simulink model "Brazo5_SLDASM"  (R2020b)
settings: Solver=VariableStepAuto  StartTime=0.0  StopTime=10.0  RelTol=1e-3
undefined symbols (not defined in the file or in its folder): deg, kg, m, N, rad, s, X, Y, Z
libraries: sm_lib x59, nesl_utility x1

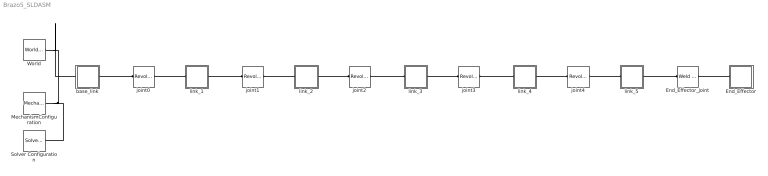
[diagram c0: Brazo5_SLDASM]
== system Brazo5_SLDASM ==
  End_Effector : Subsystem
  End_Effector_joint : sm_lib/Joints/Weld Joint  JointMode=Normal  SenseConstraintForce=off  SenseConstraintForceX=off  SenseConstraintForceY=off  SenseConstraintForceZ=off  SenseConstraintTorque=off  SenseConstraintTorqueX=off  SenseConstraintTorqueY=off  SenseConstraintTorqueZ=off  SenseTotalForce=off  SenseTotalForceX=off  SenseTotalForceY=off  SenseTotalForceZ=off  SenseTotalTorque=off  SenseTotalTorqueX=off  SenseTotalTorqueY=off  SenseTotalTorqueZ=off  CompositeWrenchDir=FollowerOnBase  CompositeWrenchFrame=BaseFrame
  MechanismConfiguration : sm_lib/Utilities/Mechanism Configuration  UniformGravity=Constant  GravityVector=[0 0 -9.80665]  GravityVectorUnits=m/s^2  GravityUnits=m/s^2  LinearizationDelta=0.001  JointModeTransitionNonlinearIterations=2
  Solver Configuration : nesl_utility/Solver Configuration  PhysicalDomain=network_engine_domain  SubClassName=solver  LeftPortType=input  RightPortType=generic  Tones=[]  Harmonics=[]  SimulateNoise=off  Profile=off  UseLocalSampling=off  EnableSwitchedLinearOptims=on  FrequencyDomain=off  UseCCode=off  RelTol=0.001  AbsTol=1e-06  MinStep=1e-09  ToWorkspace=off  RevertToSquareIcSolve=off  NumHomotopyIterations=100  PhasorMode=off  PhasorModeNumHarmonics=1  DoDC=off  ResidualTolerance=1e-09  UseLocalSolver=off  LocalSolverChoice=NE_BACKWARD_EULER_ADVANCER  LocalSolverSampleTime=0.001  DoFixedCost=off  MaxNonlinIter=3  MaxModeIter=2  ComputeImpulses=off  ImpulseIterations=2  LinearAlgebra=auto  EquationFormulation=NE_TIME_EF  DelaysMemoryBudget=1024  AutomaticFiltering=on  FilteringTimeConstant=0.001  PartitionStorageMethod=AS_NEEDED  PartitionMemoryBudget=1024  PartitionMethod=ROBUST
  World : sm_lib/Frames and Transforms/World Frame
  base_link : Subsystem
  joint0 : sm_lib/Joints/Revolute Joint  JointMode=Normal  SenseConstraintForce=off  SenseConstraintForceX=off  SenseConstraintForceY=off  SenseConstraintForceZ=off  SenseConstraintTorque=off  SenseConstraintTorqueX=off  SenseConstraintTorqueY=off  SenseConstraintTorqueZ=off  SenseTotalForce=off  SenseTotalForceX=off  SenseTotalForceY=off  SenseTotalForceZ=off  SenseTotalTorque=off  SenseTotalTorqueX=off  SenseTotalTorqueY=off  SenseTotalTorqueZ=off  CompositeWrenchDir=FollowerOnBase  CompositeWrenchFrame=BaseFrame  EquilibriumPosition=0  EquilibriumPositionUnits=deg  SpringStiffness=0  SpringStiffnessUnits=N*m/deg  DampingCoefficient=0  DampingCoefficientUnits=m^2*kg/s/rad  TorqueActuationMode=NoTorque  MotionActuationMode=ComputedMotion  SensePosition=off  SenseVelocity=off  SenseAcceleration=off  SenseTorqueForce=off  SenseLowerLimitTorqueForce=off  SenseUpperLimitTorqueForce=off  LowerLimitSpecify=on  LowerLimitBound=-2.618  LowerLimitBoundUnits=rad  LowerLimitStiffness=1e4  LowerLimitStiffnessUnits=N*m/deg  LowerLimitDamping=10  LowerLimitDampingUnits=N*m/(deg/s)  LowerLimitTransitionRegionWidth=0.1  LowerLimitTransitionRegionWidthUnits=deg  UpperLimitSpecify=on  UpperLimitBound=2.618  UpperLimitBoundUnits=rad  UpperLimitStiffness=1e4  UpperLimitStiffnessUnits=N*m/deg  UpperLimitDamping=10  UpperLimitDampingUnits=N*m/(deg/s)  UpperLimitTransitionRegionWidth=0.1  UpperLimitTransitionRegionWidthUnits=deg  PositionTargetSpecify=off  PositionTargetPriority=High  PositionTargetValue=0  PositionTargetValueUnits=deg  VelocityTargetSpecify=off  VelocityTargetPriority=High  VelocityTargetValue=0  VelocityTargetValueUnits=deg/s
  joint1 : sm_lib/Joints/Revolute Joint  JointMode=Normal  SenseConstraintForce=off  SenseConstraintForceX=off  SenseConstraintForceY=off  SenseConstraintForceZ=off  SenseConstraintTorque=off  SenseConstraintTorqueX=off  SenseConstraintTorqueY=off  SenseConstraintTorqueZ=off  SenseTotalForce=off  SenseTotalForceX=off  SenseTotalForceY=off  SenseTotalForceZ=off  SenseTotalTorque=off  SenseTotalTorqueX=off  SenseTotalTorqueY=off  SenseTotalTorqueZ=off  CompositeWrenchDir=FollowerOnBase  CompositeWrenchFrame=BaseFrame  EquilibriumPosition=0  EquilibriumPositionUnits=deg  SpringStiffness=0  SpringStiffnessUnits=N*m/deg  DampingCoefficient=0  DampingCoefficientUnits=m^2*kg/s/rad  TorqueActuationMode=NoTorque  MotionActuationMode=ComputedMotion  SensePosition=off  SenseVelocity=off  SenseAcceleration=off  SenseTorqueForce=off  SenseLowerLimitTorqueForce=off  SenseUpperLimitTorqueForce=off  LowerLimitSpecify=on  LowerLimitBound=-0.5236  LowerLimitBoundUnits=rad  LowerLimitStiffness=1e4  LowerLimitStiffnessUnits=N*m/deg  LowerLimitDamping=10  LowerLimitDampingUnits=N*m/(deg/s)  LowerLimitTransitionRegionWidth=0.1  LowerLimitTransitionRegionWidthUnits=deg  UpperLimitSpecify=on  UpperLimitBound=1.7453  UpperLimitBoundUnits=rad  UpperLimitStiffness=1e4  UpperLimitStiffnessUnits=N*m/deg  UpperLimitDamping=10  UpperLimitDampingUnits=N*m/(deg/s)  UpperLimitTransitionRegionWidth=0.1  UpperLimitTransitionRegionWidthUnits=deg  PositionTargetSpecify=off  PositionTargetPriority=High  PositionTargetValue=0  PositionTargetValueUnits=deg  VelocityTargetSpecify=off  VelocityTargetPriority=High  VelocityTargetValue=0  VelocityTargetValueUnits=deg/s
  joint2 : sm_lib/Joints/Revolute Joint  JointMode=Normal  SenseConstraintForce=off  SenseConstraintForceX=off  SenseConstraintForceY=off  SenseConstraintForceZ=off  SenseConstraintTorque=off  SenseConstraintTorqueX=off  SenseConstraintTorqueY=off  SenseConstraintTorqueZ=off  SenseTotalForce=off  SenseTotalForceX=off  SenseTotalForceY=off  SenseTotalForceZ=off  SenseTotalTorque=off  SenseTotalTorqueX=off  SenseTotalTorqueY=off  SenseTotalTorqueZ=off  CompositeWrenchDir=FollowerOnBase  CompositeWrenchFrame=BaseFrame  EquilibriumPosition=0  EquilibriumPositionUnits=deg  SpringStiffness=0  SpringStiffnessUnits=N*m/deg  DampingCoefficient=0  DampingCoefficientUnits=m^2*kg/s/rad  TorqueActuationMode=NoTorque  MotionActuationMode=ComputedMotion  SensePosition=off  SenseVelocity=off  SenseAcceleration=off  SenseTorqueForce=off  SenseLowerLimitTorqueForce=off  SenseUpperLimitTorqueForce=off  LowerLimitSpecify=on  LowerLimitBound=-0.9599  LowerLimitBoundUnits=rad  LowerLimitStiffness=1e4  LowerLimitStiffnessUnits=N*m/deg  LowerLimitDamping=10  LowerLimitDampingUnits=N*m/(deg/s)  LowerLimitTransitionRegionWidth=0.1  LowerLimitTransitionRegionWidthUnits=deg  UpperLimitSpecify=on  UpperLimitBound=0.9599  UpperLimitBoundUnits=rad  UpperLimitStiffness=1e4  UpperLimitStiffnessUnits=N*m/deg  UpperLimitDamping=10  UpperLimitDampingUnits=N*m/(deg/s)  UpperLimitTransitionRegionWidth=0.1  UpperLimitTransitionRegionWidthUnits=deg  PositionTargetSpecify=off  PositionTargetPriority=High  PositionTargetValue=0  PositionTargetValueUnits=deg  VelocityTargetSpecify=off  VelocityTargetPriority=High  VelocityTargetValue=0  VelocityTargetValueUnits=deg/s
  joint3 : sm_lib/Joints/Revolute Joint  JointMode=Normal  SenseConstraintForce=off  SenseConstraintForceX=off  SenseConstraintForceY=off  SenseConstraintForceZ=off  SenseConstraintTorque=off  SenseConstraintTorqueX=off  SenseConstraintTorqueY=off  SenseConstraintTorqueZ=off  SenseTotalForce=off  SenseTotalForceX=off  SenseTotalForceY=off  SenseTotalForceZ=off  SenseTotalTorque=off  SenseTotalTorqueX=off  SenseTotalTorqueY=off  SenseTotalTorqueZ=off  CompositeWrenchDir=FollowerOnBase  CompositeWrenchFrame=BaseFrame  EquilibriumPosition=0  EquilibriumPositionUnits=deg  SpringStiffness=0  SpringStiffnessUnits=N*m/deg  DampingCoefficient=0  DampingCoefficientUnits=m^2*kg/s/rad  TorqueActuationMode=NoTorque  MotionActuationMode=ComputedMotion  SensePosition=off  SenseVelocity=off  SenseAcceleration=off  SenseTorqueForce=off  SenseLowerLimitTorqueForce=off  SenseUpperLimitTorqueForce=off  LowerLimitSpecify=on  LowerLimitBound=-1.5708  LowerLimitBoundUnits=rad  LowerLimitStiffness=1e4  LowerLimitStiffnessUnits=N*m/deg  LowerLimitDamping=10  LowerLimitDampingUnits=N*m/(deg/s)  LowerLimitTransitionRegionWidth=0.1  LowerLimitTransitionRegionWidthUnits=deg  UpperLimitSpecify=on  UpperLimitBound=1.5708  UpperLimitBoundUnits=rad  UpperLimitStiffness=1e4  UpperLimitStiffnessUnits=N*m/deg  UpperLimitDamping=10  UpperLimitDampingUnits=N*m/(deg/s)  UpperLimitTransitionRegionWidth=0.1  UpperLimitTransitionRegionWidthUnits=deg  PositionTargetSpecify=off  PositionTargetPriority=High  PositionTargetValue=0  PositionTargetValueUnits=deg  VelocityTargetSpecify=off  VelocityTargetPriority=High  VelocityTargetValue=0  VelocityTargetValueUnits=deg/s
  joint4 : sm_lib/Joints/Revolute Joint  JointMode=Normal  SenseConstraintForce=off  SenseConstraintForceX=off  SenseConstraintForceY=off  SenseConstraintForceZ=off  SenseConstraintTorque=off  SenseConstraintTorqueX=off  SenseConstraintTorqueY=off  SenseConstraintTorqueZ=off  SenseTotalForce=off  SenseTotalForceX=off  SenseTotalForceY=off  SenseTotalForceZ=off  SenseTotalTorque=off  SenseTotalTorqueX=off  SenseTotalTorqueY=off  SenseTotalTorqueZ=off  CompositeWrenchDir=FollowerOnBase  CompositeWrenchFrame=BaseFrame  EquilibriumPosition=0  EquilibriumPositionUnits=deg  SpringStiffness=0  SpringStiffnessUnits=N*m/deg  DampingCoefficient=0  DampingCoefficientUnits=m^2*kg/s/rad  TorqueActuationMode=NoTorque  MotionActuationMode=ComputedMotion  SensePosition=off  SenseVelocity=off  SenseAcceleration=off  SenseTorqueForce=off  SenseLowerLimitTorqueForce=off  SenseUpperLimitTorqueForce=off  LowerLimitSpecify=off  LowerLimitBound=-90  LowerLimitBoundUnits=deg  LowerLimitStiffness=1e4  LowerLimitStiffnessUnits=N*m/deg  LowerLimitDamping=10  LowerLimitDampingUnits=N*m/(deg/s)  LowerLimitTransitionRegionWidth=0.1  LowerLimitTransitionRegionWidthUnits=deg  UpperLimitSpecify=off  UpperLimitBound=90  UpperLimitBoundUnits=deg  UpperLimitStiffness=1e4  UpperLimitStiffnessUnits=N*m/deg  UpperLimitDamping=10  UpperLimitDampingUnits=N*m/(deg/s)  UpperLimitTransitionRegionWidth=0.1  UpperLimitTransitionRegionWidthUnits=deg  PositionTargetSpecify=off  PositionTargetPriority=High  PositionTargetValue=0  PositionTargetValueUnits=deg  VelocityTargetSpecify=off  VelocityTargetPriority=High  VelocityTargetValue=0  VelocityTargetValueUnits=deg/s
  link_1 : Subsystem
  link_2 : Subsystem
  link_3 : Subsystem
  link_4 : Subsystem
  link_5 : Subsystem
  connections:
  End_Effector/LConn1 -- End_Effector_joint/RConn1
  base_link/RConn1 -- joint0/LConn1
  joint4/RConn1 -- link_5/LConn1
  End_Effector_joint/LConn1 -- link_5/RConn1
  World/RConn1 -- MechanismConfiguration/RConn1 -- Solver Configuration/RConn1 -- base_link/LConn1
  joint0/RConn1 -- link_1/LConn1
  joint1/LConn1 -- link_1/RConn1
  joint1/RConn1 -- link_2/LConn1
  joint2/LConn1 -- link_2/RConn1
  joint2/RConn1 -- link_3/LConn1
  joint3/LConn1 -- link_3/RConn1
  joint3/RConn1 -- link_4/LConn1
  joint4/LConn1 -- link_4/RConn1

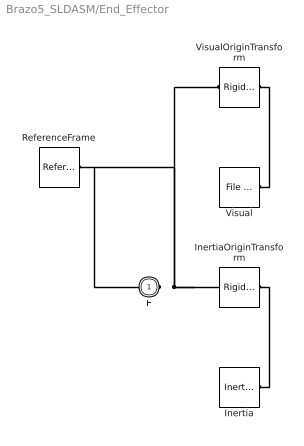
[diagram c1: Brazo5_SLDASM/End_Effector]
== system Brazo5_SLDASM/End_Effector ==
  Inertia : sm_lib/Body Elements/Inertia  InertiaType=Custom  Mass=1.4886  MassUnits=kg  CenterOfMass=[0, 0, 0]  CenterOfMassUnits=m  MomentsOfInertia=[0.00086527, 0.00086527, 0.0015073]  MomentsOfInertiaUnits=kg*m^2  ProductsOfInertia=[-1.4429e-20, -5.8421e-20, 3.3881e-21]  ProductsOfInertiaUnits=kg*m^2  GraphicType=None  MarkerShape=Inertia  MarkerSize=20  GraphicVisPropType=SimpleVisualProperties  GraphicDiffuseColor=[0.5 0.5 0.5]  GraphicSpecularColor=[0.5 0.5 0.5 1.0]  GraphicAmbientColor=[0.15 0.15 0.15 1.0]  GraphicEmissiveColor=[0.0 0.0 0.0 1.0]  GraphicShininess=75  GraphicOpacity=1.0
  InertiaOriginTransform : sm_lib/Frames and Transforms/Rigid Transform  TranslationMethod=Cartesian  TranslationStandardOffset=0  TranslationLengthUnit=m  TranslationStandardAxis=+Z  TranslationCartesianOffset=[5.5511e-17, -3.4694e-18, -0.015]  TranslationROffset=0  TranslationROffsetUnits=m  TranslationZOffset=0  TranslationZOffsetUnits=m  TranslationThetaOffset=0  TranslationThetaOffsetUnits=deg  RotationMethod=RotationSequence  RotationAngleUnits=deg  RotationStandardAxis=+Z  RotationAngle=0.0  RotationArbitraryAxis=[0 0 1]  FollAlignAxisA=+X  BaseAlignAxisA=+Y  FollAlignAxisB=+Y  BaseAlignAxisB=+Z  RotationSequenceAxes=BaseAxes  RotationSequence=XYZ  RotationSequenceAngles=[0, 0, 0]  RotationSequenceAnglesUnits=rad  RotationMatrix=[1 0 0; 0 1 0; 0 0 1]
  ReferenceFrame : sm_lib/Frames and Transforms/Reference Frame
  Visual : sm_lib/Body Elements/File Solid  ExtGeomFileName=Brazo5_SLDASM/meshes/End_Effector.STL  UnitType=Custom  ExtGeomFileUnits=m  StepReaderType=HEX  ExportConvexHullGeometry=off  InertiaType=Custom  Mass=0  MassUnits=kg  CenterOfMass=[0, 0, 0]  CenterOfMassUnits=m  MomentsOfInertia=[0, 0, 0]  MomentsOfInertiaUnits=kg*m^2  ProductsOfInertia=[0, 0, 0]  ProductsOfInertiaUnits=kg*m^2  BasedOnType=DensityFromFile  Density=1000  DensityUnits=kg/m^3  DoExposeReferenceFrame=on  SerializedFrames=<Frames/>  GraphicType=FromGeometry  MarkerShape=Sphere  MarkerSize=10  GraphicVisPropType=SimpleVisualProperties  GraphicDiffuseColor=[0.77647, 0.75686, 0.73725]  GraphicSpecularColor=[0.5 0.5 0.5 1.0]  GraphicAmbientColor=[0.15 0.15 0.15 1.0]  GraphicEmissiveColor=[0.0 0.0 0.0 1.0]  GraphicShininess=75  GraphicOpacity=1
  VisualOriginTransform : sm_lib/Frames and Transforms/Rigid Transform  TranslationMethod=Cartesian  TranslationStandardOffset=0  TranslationLengthUnit=m  TranslationStandardAxis=+Z  TranslationCartesianOffset=[0, 0, 0]  TranslationROffset=0  TranslationROffsetUnits=m  TranslationZOffset=0  TranslationZOffsetUnits=m  TranslationThetaOffset=0  TranslationThetaOffsetUnits=deg  RotationMethod=RotationSequence  RotationAngleUnits=deg  RotationStandardAxis=+Z  RotationAngle=0.0  RotationArbitraryAxis=[0 0 1]  FollAlignAxisA=+X  BaseAlignAxisA=+Y  FollAlignAxisB=+Y  BaseAlignAxisB=+Z  RotationSequenceAxes=BaseAxes  RotationSequence=XYZ  RotationSequenceAngles=[0, 0, 0]  RotationSequenceAnglesUnits=rad  RotationMatrix=[1 0 0; 0 1 0; 0 0 1]
  F : PMIOPort  Side=Left
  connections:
  Inertia/RConn1 -- InertiaOriginTransform/RConn1
  ReferenceFrame/RConn1 -- InertiaOriginTransform/LConn1 -- VisualOriginTransform/LConn1 -- F/RConn1
  Visual/RConn1 -- VisualOriginTransform/RConn1

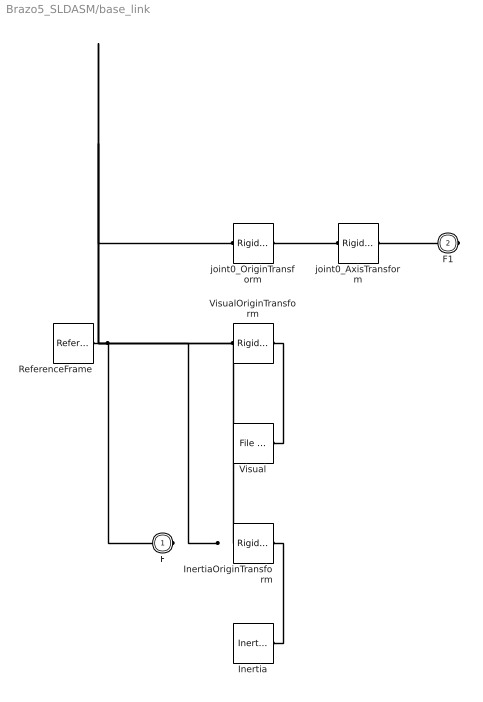
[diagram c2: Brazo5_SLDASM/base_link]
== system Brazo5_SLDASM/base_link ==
  Inertia : sm_lib/Body Elements/Inertia  InertiaType=Custom  Mass=24.7510397618277  MassUnits=kg  CenterOfMass=[0, 0, 0]  CenterOfMassUnits=m  MomentsOfInertia=[0.0874801756562005, 0.0874759059101369, 0.08538874734227481]  MomentsOfInertiaUnits=kg*m^2  ProductsOfInertia=[9.227257706190509e-08, 1.66550942408297e-07, -1.07699296841389e-07]  ProductsOfInertiaUnits=kg*m^2  GraphicType=None  MarkerShape=Inertia  MarkerSize=20  GraphicVisPropType=SimpleVisualProperties  GraphicDiffuseColor=[0.5 0.5 0.5]  GraphicSpecularColor=[0.5 0.5 0.5 1.0]  GraphicAmbientColor=[0.15 0.15 0.15 1.0]  GraphicEmissiveColor=[0.0 0.0 0.0 1.0]  GraphicShininess=75  GraphicOpacity=1.0
  InertiaOriginTransform : sm_lib/Frames and Transforms/Rigid Transform  TranslationMethod=Cartesian  TranslationStandardOffset=0  TranslationLengthUnit=m  TranslationStandardAxis=+Z  TranslationCartesianOffset=[-3.38903049823907e-08, 1.11389311641252e-06, 0.0695274745393441]  TranslationROffset=0  TranslationROffsetUnits=m  TranslationZOffset=0  TranslationZOffsetUnits=m  TranslationThetaOffset=0  TranslationThetaOffsetUnits=deg  RotationMethod=RotationSequence  RotationAngleUnits=deg  RotationStandardAxis=+Z  RotationAngle=0.0  RotationArbitraryAxis=[0 0 1]  FollAlignAxisA=+X  BaseAlignAxisA=+Y  FollAlignAxisB=+Y  BaseAlignAxisB=+Z  RotationSequenceAxes=BaseAxes  RotationSequence=XYZ  RotationSequenceAngles=[0, 0, 0]  RotationSequenceAnglesUnits=rad  RotationMatrix=[1 0 0; 0 1 0; 0 0 1]
  ReferenceFrame : sm_lib/Frames and Transforms/Reference Frame
  Visual : sm_lib/Body Elements/File Solid  ExtGeomFileName=Brazo5_SLDASM/meshes/base_link.STL  UnitType=Custom  ExtGeomFileUnits=m  StepReaderType=HEX  ExportConvexHullGeometry=off  InertiaType=Custom  Mass=0  MassUnits=kg  CenterOfMass=[0, 0, 0]  CenterOfMassUnits=m  MomentsOfInertia=[0, 0, 0]  MomentsOfInertiaUnits=kg*m^2  ProductsOfInertia=[0, 0, 0]  ProductsOfInertiaUnits=kg*m^2  BasedOnType=DensityFromFile  Density=1000  DensityUnits=kg/m^3  DoExposeReferenceFrame=on  SerializedFrames=<Frames/>  GraphicType=FromGeometry  MarkerShape=Sphere  MarkerSize=10  GraphicVisPropType=SimpleVisualProperties  GraphicDiffuseColor=[0.776470588235294, 0.756862745098039, 0.737254901960784]  GraphicSpecularColor=[0.5 0.5 0.5 1.0]  GraphicAmbientColor=[0.15 0.15 0.15 1.0]  GraphicEmissiveColor=[0.0 0.0 0.0 1.0]  GraphicShininess=75  GraphicOpacity=1
  VisualOriginTransform : sm_lib/Frames and Transforms/Rigid Transform  TranslationMethod=Cartesian  TranslationStandardOffset=0  TranslationLengthUnit=m  TranslationStandardAxis=+Z  TranslationCartesianOffset=[0, 0, 0]  TranslationROffset=0  TranslationROffsetUnits=m  TranslationZOffset=0  TranslationZOffsetUnits=m  TranslationThetaOffset=0  TranslationThetaOffsetUnits=deg  RotationMethod=RotationSequence  RotationAngleUnits=deg  RotationStandardAxis=+Z  RotationAngle=0.0  RotationArbitraryAxis=[0 0 1]  FollAlignAxisA=+X  BaseAlignAxisA=+Y  FollAlignAxisB=+Y  BaseAlignAxisB=+Z  RotationSequenceAxes=BaseAxes  RotationSequence=XYZ  RotationSequenceAngles=[0, 0, 0]  RotationSequenceAnglesUnits=rad  RotationMatrix=[1 0 0; 0 1 0; 0 0 1]
  joint0_AxisTransform : sm_lib/Frames and Transforms/Rigid Transform  TranslationMethod=Cartesian  TranslationStandardOffset=0  TranslationLengthUnit=m  TranslationStandardAxis=+Z  TranslationCartesianOffset=[0, 0, 0]  TranslationROffset=0  TranslationROffsetUnits=m  TranslationZOffset=0  TranslationZOffsetUnits=m  TranslationThetaOffset=0  TranslationThetaOffsetUnits=deg  RotationMethod=ArbitraryAxis  RotationAngleUnits=rad  RotationStandardAxis=+Z  RotationAngle=0  RotationArbitraryAxis=[1, 0, 0]  FollAlignAxisA=+X  BaseAlignAxisA=+Y  FollAlignAxisB=+Y  BaseAlignAxisB=+Z  RotationSequenceAxes=FollowerAxes  RotationSequence=XYX  RotationSequenceAngles=[0 0 0]  RotationSequenceAnglesUnits=deg  RotationMatrix=[1 0 0; 0 1 0; 0 0 1]
  joint0_OriginTransform : sm_lib/Frames and Transforms/Rigid Transform  TranslationMethod=Cartesian  TranslationStandardOffset=0  TranslationLengthUnit=m  TranslationStandardAxis=+Z  TranslationCartesianOffset=[0, 0, 0]  TranslationROffset=0  TranslationROffsetUnits=m  TranslationZOffset=0  TranslationZOffsetUnits=m  TranslationThetaOffset=0  TranslationThetaOffsetUnits=deg  RotationMethod=RotationSequence  RotationAngleUnits=deg  RotationStandardAxis=+Z  RotationAngle=0.0  RotationArbitraryAxis=[0 0 1]  FollAlignAxisA=+X  BaseAlignAxisA=+Y  FollAlignAxisB=+Y  BaseAlignAxisB=+Z  RotationSequenceAxes=BaseAxes  RotationSequence=XYZ  RotationSequenceAngles=[0, 0, 0]  RotationSequenceAnglesUnits=rad  RotationMatrix=[1 0 0; 0 1 0; 0 0 1]
  F : PMIOPort  Side=Left
  F1 : PMIOPort  Port=2  Side=Right
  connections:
  Inertia/RConn1 -- InertiaOriginTransform/RConn1
  ReferenceFrame/RConn1 -- InertiaOriginTransform/LConn1 -- VisualOriginTransform/LConn1 -- joint0_OriginTransform/LConn1 -- F/RConn1
  Visual/RConn1 -- VisualOriginTransform/RConn1
  joint0_AxisTransform/RConn1 -- F1/RConn1
  joint0_AxisTransform/LConn1 -- joint0_OriginTransform/RConn1

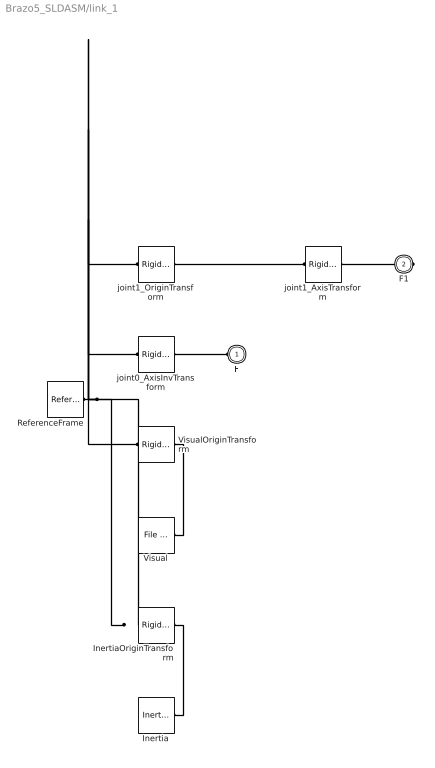
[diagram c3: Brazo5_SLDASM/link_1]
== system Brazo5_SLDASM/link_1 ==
  Inertia : sm_lib/Body Elements/Inertia  InertiaType=Custom  Mass=40.0845288402432  MassUnits=kg  CenterOfMass=[0, 0, 0]  CenterOfMassUnits=m  MomentsOfInertia=[0.14010759767158, 0.151242200998818, 0.165885928760033]  MomentsOfInertiaUnits=kg*m^2  ProductsOfInertia=[-5.20692886539246e-17, 1.32894629589073e-17, 1.5890318187219e-18]  ProductsOfInertiaUnits=kg*m^2  GraphicType=None  MarkerShape=Inertia  MarkerSize=20  GraphicVisPropType=SimpleVisualProperties  GraphicDiffuseColor=[0.5 0.5 0.5]  GraphicSpecularColor=[0.5 0.5 0.5 1.0]  GraphicAmbientColor=[0.15 0.15 0.15 1.0]  GraphicEmissiveColor=[0.0 0.0 0.0 1.0]  GraphicShininess=75  GraphicOpacity=1.0
  InertiaOriginTransform : sm_lib/Frames and Transforms/Rigid Transform  TranslationMethod=Cartesian  TranslationStandardOffset=0  TranslationLengthUnit=m  TranslationStandardAxis=+Z  TranslationCartesianOffset=[2.24939232534553e-17, 2.46845186444496e-06, 0.28325146066136]  TranslationROffset=0  TranslationROffsetUnits=m  TranslationZOffset=0  TranslationZOffsetUnits=m  TranslationThetaOffset=0  TranslationThetaOffsetUnits=deg  RotationMethod=RotationSequence  RotationAngleUnits=deg  RotationStandardAxis=+Z  RotationAngle=0.0  RotationArbitraryAxis=[0 0 1]  FollAlignAxisA=+X  BaseAlignAxisA=+Y  FollAlignAxisB=+Y  BaseAlignAxisB=+Z  RotationSequenceAxes=BaseAxes  RotationSequence=XYZ  RotationSequenceAngles=[0, 0, 0]  RotationSequenceAnglesUnits=rad  RotationMatrix=[1 0 0; 0 1 0; 0 0 1]
  ReferenceFrame : sm_lib/Frames and Transforms/Reference Frame
  Visual : sm_lib/Body Elements/File Solid  ExtGeomFileName=Brazo5_SLDASM/meshes/link_1.STL  UnitType=Custom  ExtGeomFileUnits=m  StepReaderType=HEX  ExportConvexHullGeometry=off  InertiaType=Custom  Mass=0  MassUnits=kg  CenterOfMass=[0, 0, 0]  CenterOfMassUnits=m  MomentsOfInertia=[0, 0, 0]  MomentsOfInertiaUnits=kg*m^2  ProductsOfInertia=[0, 0, 0]  ProductsOfInertiaUnits=kg*m^2  BasedOnType=DensityFromFile  Density=1000  DensityUnits=kg/m^3  DoExposeReferenceFrame=on  SerializedFrames=<Frames/>  GraphicType=FromGeometry  MarkerShape=Sphere  MarkerSize=10  GraphicVisPropType=SimpleVisualProperties  GraphicDiffuseColor=[0.776470588235294, 0.756862745098039, 0.737254901960784]  GraphicSpecularColor=[0.5 0.5 0.5 1.0]  GraphicAmbientColor=[0.15 0.15 0.15 1.0]  GraphicEmissiveColor=[0.0 0.0 0.0 1.0]  GraphicShininess=75  GraphicOpacity=1
  VisualOriginTransform : sm_lib/Frames and Transforms/Rigid Transform  TranslationMethod=Cartesian  TranslationStandardOffset=0  TranslationLengthUnit=m  TranslationStandardAxis=+Z  TranslationCartesianOffset=[0, 0, 0]  TranslationROffset=0  TranslationROffsetUnits=m  TranslationZOffset=0  TranslationZOffsetUnits=m  TranslationThetaOffset=0  TranslationThetaOffsetUnits=deg  RotationMethod=RotationSequence  RotationAngleUnits=deg  RotationStandardAxis=+Z  RotationAngle=0.0  RotationArbitraryAxis=[0 0 1]  FollAlignAxisA=+X  BaseAlignAxisA=+Y  FollAlignAxisB=+Y  BaseAlignAxisB=+Z  RotationSequenceAxes=BaseAxes  RotationSequence=XYZ  RotationSequenceAngles=[0, 0, 0]  RotationSequenceAnglesUnits=rad  RotationMatrix=[1 0 0; 0 1 0; 0 0 1]
  joint0_AxisInvTransform : sm_lib/Frames and Transforms/Rigid Transform  TranslationMethod=Cartesian  TranslationStandardOffset=0  TranslationLengthUnit=m  TranslationStandardAxis=+Z  TranslationCartesianOffset=[0, 0, 0]  TranslationROffset=0  TranslationROffsetUnits=m  TranslationZOffset=0  TranslationZOffsetUnits=m  TranslationThetaOffset=0  TranslationThetaOffsetUnits=deg  RotationMethod=ArbitraryAxis  RotationAngleUnits=rad  RotationStandardAxis=+Z  RotationAngle=0  RotationArbitraryAxis=[1, 0, 0]  FollAlignAxisA=+X  BaseAlignAxisA=+Y  FollAlignAxisB=+Y  BaseAlignAxisB=+Z  RotationSequenceAxes=FollowerAxes  RotationSequence=XYX  RotationSequenceAngles=[0 0 0]  RotationSequenceAnglesUnits=deg  RotationMatrix=[1 0 0; 0 1 0; 0 0 1]
  joint1_AxisTransform : sm_lib/Frames and Transforms/Rigid Transform  TranslationMethod=Cartesian  TranslationStandardOffset=0  TranslationLengthUnit=m  TranslationStandardAxis=+Z  TranslationCartesianOffset=[0, 0, 0]  TranslationROffset=0  TranslationROffsetUnits=m  TranslationZOffset=0  TranslationZOffsetUnits=m  TranslationThetaOffset=0  TranslationThetaOffsetUnits=deg  RotationMethod=ArbitraryAxis  RotationAngleUnits=rad  RotationStandardAxis=+Z  RotationAngle=0  RotationArbitraryAxis=[1, 0, 0]  FollAlignAxisA=+X  BaseAlignAxisA=+Y  FollAlignAxisB=+Y  BaseAlignAxisB=+Z  RotationSequenceAxes=FollowerAxes  RotationSequence=XYX  RotationSequenceAngles=[0 0 0]  RotationSequenceAnglesUnits=deg  RotationMatrix=[1 0 0; 0 1 0; 0 0 1]
  joint1_OriginTransform : sm_lib/Frames and Transforms/Rigid Transform  TranslationMethod=Cartesian  TranslationStandardOffset=0  TranslationLengthUnit=m  TranslationStandardAxis=+Z  TranslationCartesianOffset=[0, 0, 0.35051]  TranslationROffset=0  TranslationROffsetUnits=m  TranslationZOffset=0  TranslationZOffsetUnits=m  TranslationThetaOffset=0  TranslationThetaOffsetUnits=deg  RotationMethod=RotationSequence  RotationAngleUnits=deg  RotationStandardAxis=+Z  RotationAngle=0.0  RotationArbitraryAxis=[0 0 1]  FollAlignAxisA=+X  BaseAlignAxisA=+Y  FollAlignAxisB=+Y  BaseAlignAxisB=+Z  RotationSequenceAxes=BaseAxes  RotationSequence=XYZ  RotationSequenceAngles=[1.5708, 0, 1.5708]  RotationSequenceAnglesUnits=rad  RotationMatrix=[1 0 0; 0 1 0; 0 0 1]
  F : PMIOPort  Side=Left
  F1 : PMIOPort  Port=2  Side=Right
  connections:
  Inertia/RConn1 -- InertiaOriginTransform/RConn1
  ReferenceFrame/RConn1 -- InertiaOriginTransform/LConn1 -- VisualOriginTransform/LConn1 -- joint0_AxisInvTransform/LConn1 -- joint1_OriginTransform/LConn1
  Visual/RConn1 -- VisualOriginTransform/RConn1
  joint0_AxisInvTransform/RConn1 -- F/RConn1
  joint1_AxisTransform/RConn1 -- F1/RConn1
  joint1_AxisTransform/LConn1 -- joint1_OriginTransform/RConn1

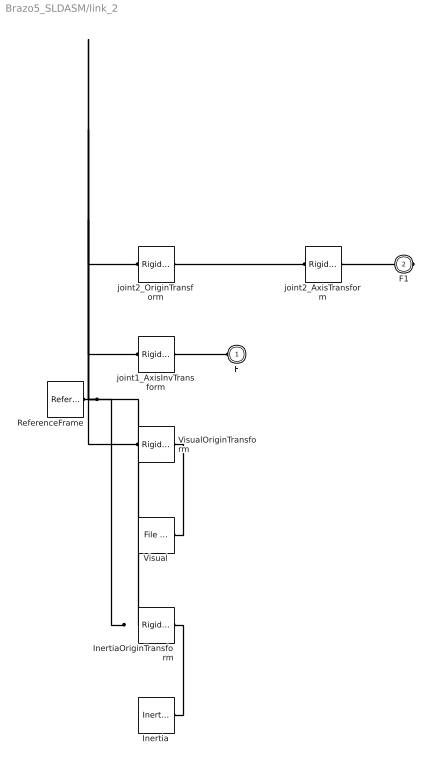
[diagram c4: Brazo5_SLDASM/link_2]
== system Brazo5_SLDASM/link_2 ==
  Inertia : sm_lib/Body Elements/Inertia  InertiaType=Custom  Mass=34.1892669715201  MassUnits=kg  CenterOfMass=[0, 0, 0]  CenterOfMassUnits=m  MomentsOfInertia=[0.100999689869813, 0.323464785078339, 0.28584252374745]  MomentsOfInertiaUnits=kg*m^2  ProductsOfInertia=[-2.19096219704951e-18, 8.5802322320121e-17, 3.73980846905113e-17]  ProductsOfInertiaUnits=kg*m^2  GraphicType=None  MarkerShape=Inertia  MarkerSize=20  GraphicVisPropType=SimpleVisualProperties  GraphicDiffuseColor=[0.5 0.5 0.5]  GraphicSpecularColor=[0.5 0.5 0.5 1.0]  GraphicAmbientColor=[0.15 0.15 0.15 1.0]  GraphicEmissiveColor=[0.0 0.0 0.0 1.0]  GraphicShininess=75  GraphicOpacity=1.0
  InertiaOriginTransform : sm_lib/Frames and Transforms/Rigid Transform  TranslationMethod=Cartesian  TranslationStandardOffset=0  TranslationLengthUnit=m  TranslationStandardAxis=+Z  TranslationCartesianOffset=[0.07391242231991781, 0, -1.2931997966502e-17]  TranslationROffset=0  TranslationROffsetUnits=m  TranslationZOffset=0  TranslationZOffsetUnits=m  TranslationThetaOffset=0  TranslationThetaOffsetUnits=deg  RotationMethod=RotationSequence  RotationAngleUnits=deg  RotationStandardAxis=+Z  RotationAngle=0.0  RotationArbitraryAxis=[0 0 1]  FollAlignAxisA=+X  BaseAlignAxisA=+Y  FollAlignAxisB=+Y  BaseAlignAxisB=+Z  RotationSequenceAxes=BaseAxes  RotationSequence=XYZ  RotationSequenceAngles=[0, 0, 0]  RotationSequenceAnglesUnits=rad  RotationMatrix=[1 0 0; 0 1 0; 0 0 1]
  ReferenceFrame : sm_lib/Frames and Transforms/Reference Frame
  Visual : sm_lib/Body Elements/File Solid  ExtGeomFileName=Brazo5_SLDASM/meshes/link_2.STL  UnitType=Custom  ExtGeomFileUnits=m  StepReaderType=HEX  ExportConvexHullGeometry=off  InertiaType=Custom  Mass=0  MassUnits=kg  CenterOfMass=[0, 0, 0]  CenterOfMassUnits=m  MomentsOfInertia=[0, 0, 0]  MomentsOfInertiaUnits=kg*m^2  ProductsOfInertia=[0, 0, 0]  ProductsOfInertiaUnits=kg*m^2  BasedOnType=DensityFromFile  Density=1000  DensityUnits=kg/m^3  DoExposeReferenceFrame=on  SerializedFrames=<Frames/>  GraphicType=FromGeometry  MarkerShape=Sphere  MarkerSize=10  GraphicVisPropType=SimpleVisualProperties  GraphicDiffuseColor=[0.776470588235294, 0.756862745098039, 0.737254901960784]  GraphicSpecularColor=[0.5 0.5 0.5 1.0]  GraphicAmbientColor=[0.15 0.15 0.15 1.0]  GraphicEmissiveColor=[0.0 0.0 0.0 1.0]  GraphicShininess=75  GraphicOpacity=1
  VisualOriginTransform : sm_lib/Frames and Transforms/Rigid Transform  TranslationMethod=Cartesian  TranslationStandardOffset=0  TranslationLengthUnit=m  TranslationStandardAxis=+Z  TranslationCartesianOffset=[0, 0, 0]  TranslationROffset=0  TranslationROffsetUnits=m  TranslationZOffset=0  TranslationZOffsetUnits=m  TranslationThetaOffset=0  TranslationThetaOffsetUnits=deg  RotationMethod=RotationSequence  RotationAngleUnits=deg  RotationStandardAxis=+Z  RotationAngle=0.0  RotationArbitraryAxis=[0 0 1]  FollAlignAxisA=+X  BaseAlignAxisA=+Y  FollAlignAxisB=+Y  BaseAlignAxisB=+Z  RotationSequenceAxes=BaseAxes  RotationSequence=XYZ  RotationSequenceAngles=[0, 0, 0]  RotationSequenceAnglesUnits=rad  RotationMatrix=[1 0 0; 0 1 0; 0 0 1]
  joint1_AxisInvTransform : sm_lib/Frames and Transforms/Rigid Transform  TranslationMethod=Cartesian  TranslationStandardOffset=0  TranslationLengthUnit=m  TranslationStandardAxis=+Z  TranslationCartesianOffset=[0, 0, 0]  TranslationROffset=0  TranslationROffsetUnits=m  TranslationZOffset=0  TranslationZOffsetUnits=m  TranslationThetaOffset=0  TranslationThetaOffsetUnits=deg  RotationMethod=ArbitraryAxis  RotationAngleUnits=rad  RotationStandardAxis=+Z  RotationAngle=0  RotationArbitraryAxis=[1, 0, 0]  FollAlignAxisA=+X  BaseAlignAxisA=+Y  FollAlignAxisB=+Y  BaseAlignAxisB=+Z  RotationSequenceAxes=FollowerAxes  RotationSequence=XYX  RotationSequenceAngles=[0 0 0]  RotationSequenceAnglesUnits=deg  RotationMatrix=[1 0 0; 0 1 0; 0 0 1]
  joint2_AxisTransform : sm_lib/Frames and Transforms/Rigid Transform  TranslationMethod=Cartesian  TranslationStandardOffset=0  TranslationLengthUnit=m  TranslationStandardAxis=+Z  TranslationCartesianOffset=[0, 0, 0]  TranslationROffset=0  TranslationROffsetUnits=m  TranslationZOffset=0  TranslationZOffsetUnits=m  TranslationThetaOffset=0  TranslationThetaOffsetUnits=deg  RotationMethod=ArbitraryAxis  RotationAngleUnits=rad  RotationStandardAxis=+Z  RotationAngle=0  RotationArbitraryAxis=[1, 0, 0]  FollAlignAxisA=+X  BaseAlignAxisA=+Y  FollAlignAxisB=+Y  BaseAlignAxisB=+Z  RotationSequenceAxes=FollowerAxes  RotationSequence=XYX  RotationSequenceAngles=[0 0 0]  RotationSequenceAnglesUnits=deg  RotationMatrix=[1 0 0; 0 1 0; 0 0 1]
  joint2_OriginTransform : sm_lib/Frames and Transforms/Rigid Transform  TranslationMethod=Cartesian  TranslationStandardOffset=0  TranslationLengthUnit=m  TranslationStandardAxis=+Z  TranslationCartesianOffset=[0.25, 0, 0]  TranslationROffset=0  TranslationROffsetUnits=m  TranslationZOffset=0  TranslationZOffsetUnits=m  TranslationThetaOffset=0  TranslationThetaOffsetUnits=deg  RotationMethod=RotationSequence  RotationAngleUnits=deg  RotationStandardAxis=+Z  RotationAngle=0.0  RotationArbitraryAxis=[0 0 1]  FollAlignAxisA=+X  BaseAlignAxisA=+Y  FollAlignAxisB=+Y  BaseAlignAxisB=+Z  RotationSequenceAxes=BaseAxes  RotationSequence=XYZ  RotationSequenceAngles=[0, 0, 0]  RotationSequenceAnglesUnits=rad  RotationMatrix=[1 0 0; 0 1 0; 0 0 1]
  F : PMIOPort  Side=Left
  F1 : PMIOPort  Port=2  Side=Right
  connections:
  Inertia/RConn1 -- InertiaOriginTransform/RConn1
  ReferenceFrame/RConn1 -- InertiaOriginTransform/LConn1 -- VisualOriginTransform/LConn1 -- joint1_AxisInvTransform/LConn1 -- joint2_OriginTransform/LConn1
  Visual/RConn1 -- VisualOriginTransform/RConn1
  joint1_AxisInvTransform/RConn1 -- F/RConn1
  joint2_AxisTransform/RConn1 -- F1/RConn1
  joint2_AxisTransform/LConn1 -- joint2_OriginTransform/RConn1

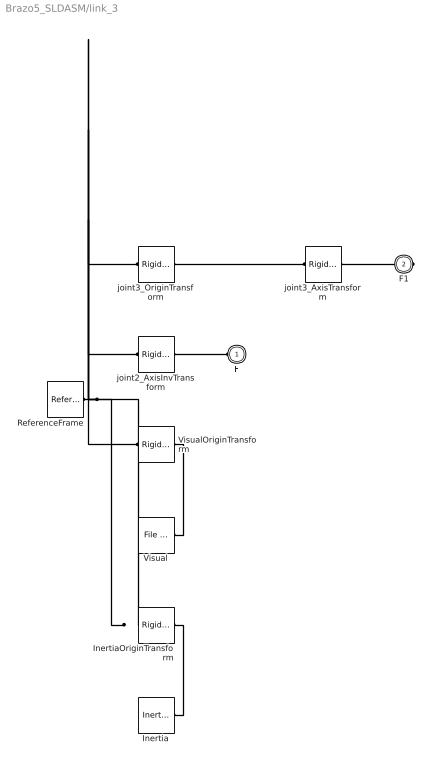
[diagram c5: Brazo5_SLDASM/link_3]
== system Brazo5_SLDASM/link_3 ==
  Inertia : sm_lib/Body Elements/Inertia  InertiaType=Custom  Mass=13.9460998385185  MassUnits=kg  CenterOfMass=[0, 0, 0]  CenterOfMassUnits=m  MomentsOfInertia=[0.026465483583986, 0.0628137115265308, 0.0543358776965413]  MomentsOfInertiaUnits=kg*m^2  ProductsOfInertia=[-5.14627121152742e-19, 1.96375333381757e-17, 6.41551043751981e-18]  ProductsOfInertiaUnits=kg*m^2  GraphicType=None  MarkerShape=Inertia  MarkerSize=20  GraphicVisPropType=SimpleVisualProperties  GraphicDiffuseColor=[0.5 0.5 0.5]  GraphicSpecularColor=[0.5 0.5 0.5 1.0]  GraphicAmbientColor=[0.15 0.15 0.15 1.0]  GraphicEmissiveColor=[0.0 0.0 0.0 1.0]  GraphicShininess=75  GraphicOpacity=1.0
  InertiaOriginTransform : sm_lib/Frames and Transforms/Rigid Transform  TranslationMethod=Cartesian  TranslationStandardOffset=0  TranslationLengthUnit=m  TranslationStandardAxis=+Z  TranslationCartesianOffset=[0.0538405076409555, 0, -2.89254125393904e-17]  TranslationROffset=0  TranslationROffsetUnits=m  TranslationZOffset=0  TranslationZOffsetUnits=m  TranslationThetaOffset=0  TranslationThetaOffsetUnits=deg  RotationMethod=RotationSequence  RotationAngleUnits=deg  RotationStandardAxis=+Z  RotationAngle=0.0  RotationArbitraryAxis=[0 0 1]  FollAlignAxisA=+X  BaseAlignAxisA=+Y  FollAlignAxisB=+Y  BaseAlignAxisB=+Z  RotationSequenceAxes=BaseAxes  RotationSequence=XYZ  RotationSequenceAngles=[0, 0, 0]  RotationSequenceAnglesUnits=rad  RotationMatrix=[1 0 0; 0 1 0; 0 0 1]
  ReferenceFrame : sm_lib/Frames and Transforms/Reference Frame
  Visual : sm_lib/Body Elements/File Solid  ExtGeomFileName=Brazo5_SLDASM/meshes/link_3.STL  UnitType=Custom  ExtGeomFileUnits=m  StepReaderType=HEX  ExportConvexHullGeometry=off  InertiaType=Custom  Mass=0  MassUnits=kg  CenterOfMass=[0, 0, 0]  CenterOfMassUnits=m  MomentsOfInertia=[0, 0, 0]  MomentsOfInertiaUnits=kg*m^2  ProductsOfInertia=[0, 0, 0]  ProductsOfInertiaUnits=kg*m^2  BasedOnType=DensityFromFile  Density=1000  DensityUnits=kg/m^3  DoExposeReferenceFrame=on  SerializedFrames=<Frames/>  GraphicType=FromGeometry  MarkerShape=Sphere  MarkerSize=10  GraphicVisPropType=SimpleVisualProperties  GraphicDiffuseColor=[0.776470588235294, 0.756862745098039, 0.737254901960784]  GraphicSpecularColor=[0.5 0.5 0.5 1.0]  GraphicAmbientColor=[0.15 0.15 0.15 1.0]  GraphicEmissiveColor=[0.0 0.0 0.0 1.0]  GraphicShininess=75  GraphicOpacity=1
  VisualOriginTransform : sm_lib/Frames and Transforms/Rigid Transform  TranslationMethod=Cartesian  TranslationStandardOffset=0  TranslationLengthUnit=m  TranslationStandardAxis=+Z  TranslationCartesianOffset=[0, 0, 0]  TranslationROffset=0  TranslationROffsetUnits=m  TranslationZOffset=0  TranslationZOffsetUnits=m  TranslationThetaOffset=0  TranslationThetaOffsetUnits=deg  RotationMethod=RotationSequence  RotationAngleUnits=deg  RotationStandardAxis=+Z  RotationAngle=0.0  RotationArbitraryAxis=[0 0 1]  FollAlignAxisA=+X  BaseAlignAxisA=+Y  FollAlignAxisB=+Y  BaseAlignAxisB=+Z  RotationSequenceAxes=BaseAxes  RotationSequence=XYZ  RotationSequenceAngles=[0, 0, 0]  RotationSequenceAnglesUnits=rad  RotationMatrix=[1 0 0; 0 1 0; 0 0 1]
  joint2_AxisInvTransform : sm_lib/Frames and Transforms/Rigid Transform  TranslationMethod=Cartesian  TranslationStandardOffset=0  TranslationLengthUnit=m  TranslationStandardAxis=+Z  TranslationCartesianOffset=[0, 0, 0]  TranslationROffset=0  TranslationROffsetUnits=m  TranslationZOffset=0  TranslationZOffsetUnits=m  TranslationThetaOffset=0  TranslationThetaOffsetUnits=deg  RotationMethod=ArbitraryAxis  RotationAngleUnits=rad  RotationStandardAxis=+Z  RotationAngle=0  RotationArbitraryAxis=[1, 0, 0]  FollAlignAxisA=+X  BaseAlignAxisA=+Y  FollAlignAxisB=+Y  BaseAlignAxisB=+Z  RotationSequenceAxes=FollowerAxes  RotationSequence=XYX  RotationSequenceAngles=[0 0 0]  RotationSequenceAnglesUnits=deg  RotationMatrix=[1 0 0; 0 1 0; 0 0 1]
  joint3_AxisTransform : sm_lib/Frames and Transforms/Rigid Transform  TranslationMethod=Cartesian  TranslationStandardOffset=0  TranslationLengthUnit=m  TranslationStandardAxis=+Z  TranslationCartesianOffset=[0, 0, 0]  TranslationROffset=0  TranslationROffsetUnits=m  TranslationZOffset=0  TranslationZOffsetUnits=m  TranslationThetaOffset=0  TranslationThetaOffsetUnits=deg  RotationMethod=ArbitraryAxis  RotationAngleUnits=rad  RotationStandardAxis=+Z  RotationAngle=0  RotationArbitraryAxis=[1, 0, 0]  FollAlignAxisA=+X  BaseAlignAxisA=+Y  FollAlignAxisB=+Y  BaseAlignAxisB=+Z  RotationSequenceAxes=FollowerAxes  RotationSequence=XYX  RotationSequenceAngles=[0 0 0]  RotationSequenceAnglesUnits=deg  RotationMatrix=[1 0 0; 0 1 0; 0 0 1]
  joint3_OriginTransform : sm_lib/Frames and Transforms/Rigid Transform  TranslationMethod=Cartesian  TranslationStandardOffset=0  TranslationLengthUnit=m  TranslationStandardAxis=+Z  TranslationCartesianOffset=[0.16, 0, 0]  TranslationROffset=0  TranslationROffsetUnits=m  TranslationZOffset=0  TranslationZOffsetUnits=m  TranslationThetaOffset=0  TranslationThetaOffsetUnits=deg  RotationMethod=RotationSequence  RotationAngleUnits=deg  RotationStandardAxis=+Z  RotationAngle=0.0  RotationArbitraryAxis=[0 0 1]  FollAlignAxisA=+X  BaseAlignAxisA=+Y  FollAlignAxisB=+Y  BaseAlignAxisB=+Z  RotationSequenceAxes=BaseAxes  RotationSequence=XYZ  RotationSequenceAngles=[0, 0, 0]  RotationSequenceAnglesUnits=rad  RotationMatrix=[1 0 0; 0 1 0; 0 0 1]
  F : PMIOPort  Side=Left
  F1 : PMIOPort  Port=2  Side=Right
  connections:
  Inertia/RConn1 -- InertiaOriginTransform/RConn1
  ReferenceFrame/RConn1 -- InertiaOriginTransform/LConn1 -- VisualOriginTransform/LConn1 -- joint2_AxisInvTransform/LConn1 -- joint3_OriginTransform/LConn1
  Visual/RConn1 -- VisualOriginTransform/RConn1
  joint2_AxisInvTransform/RConn1 -- F/RConn1
  joint3_AxisTransform/RConn1 -- F1/RConn1
  joint3_AxisTransform/LConn1 -- joint3_OriginTransform/RConn1

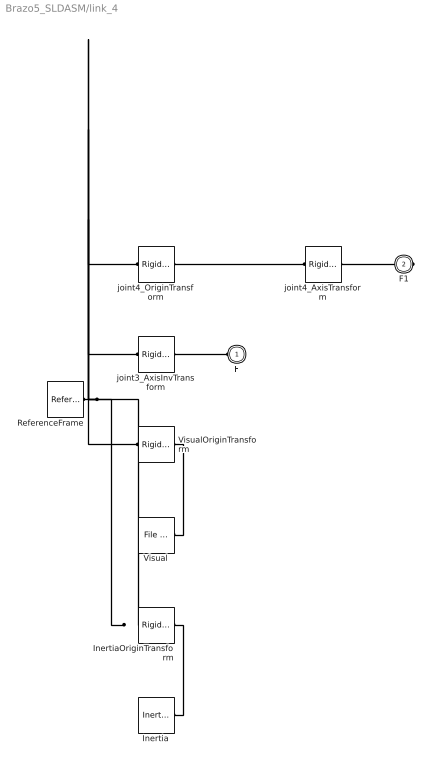
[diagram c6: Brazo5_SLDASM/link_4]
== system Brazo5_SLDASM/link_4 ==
  Inertia : sm_lib/Body Elements/Inertia  InertiaType=Custom  Mass=2.62582123658694  MassUnits=kg  CenterOfMass=[0, 0, 0]  CenterOfMassUnits=m  MomentsOfInertia=[0.00197083600155281, 0.00325865261538323, 0.00214733918833594]  MomentsOfInertiaUnits=kg*m^2  ProductsOfInertia=[-1.26269021628898e-19, -3.10811231220588e-19, 2.23060660101183e-20]  ProductsOfInertiaUnits=kg*m^2  GraphicType=None  MarkerShape=Inertia  MarkerSize=20  GraphicVisPropType=SimpleVisualProperties  GraphicDiffuseColor=[0.5 0.5 0.5]  GraphicSpecularColor=[0.5 0.5 0.5 1.0]  GraphicAmbientColor=[0.15 0.15 0.15 1.0]  GraphicEmissiveColor=[0.0 0.0 0.0 1.0]  GraphicShininess=75  GraphicOpacity=1.0
  InertiaOriginTransform : sm_lib/Frames and Transforms/Rigid Transform  TranslationMethod=Cartesian  TranslationStandardOffset=0  TranslationLengthUnit=m  TranslationStandardAxis=+Z  TranslationCartesianOffset=[0.0260264378448915, -5.55111512312578e-17, 3.20676455869593e-17]  TranslationROffset=0  TranslationROffsetUnits=m  TranslationZOffset=0  TranslationZOffsetUnits=m  TranslationThetaOffset=0  TranslationThetaOffsetUnits=deg  RotationMethod=RotationSequence  RotationAngleUnits=deg  RotationStandardAxis=+Z  RotationAngle=0.0  RotationArbitraryAxis=[0 0 1]  FollAlignAxisA=+X  BaseAlignAxisA=+Y  FollAlignAxisB=+Y  BaseAlignAxisB=+Z  RotationSequenceAxes=BaseAxes  RotationSequence=XYZ  RotationSequenceAngles=[0, 0, 0]  RotationSequenceAnglesUnits=rad  RotationMatrix=[1 0 0; 0 1 0; 0 0 1]
  ReferenceFrame : sm_lib/Frames and Transforms/Reference Frame
  Visual : sm_lib/Body Elements/File Solid  ExtGeomFileName=Brazo5_SLDASM/meshes/link_4.STL  UnitType=Custom  ExtGeomFileUnits=m  StepReaderType=HEX  ExportConvexHullGeometry=off  InertiaType=Custom  Mass=0  MassUnits=kg  CenterOfMass=[0, 0, 0]  CenterOfMassUnits=m  MomentsOfInertia=[0, 0, 0]  MomentsOfInertiaUnits=kg*m^2  ProductsOfInertia=[0, 0, 0]  ProductsOfInertiaUnits=kg*m^2  BasedOnType=DensityFromFile  Density=1000  DensityUnits=kg/m^3  DoExposeReferenceFrame=on  SerializedFrames=<Frames/>  GraphicType=FromGeometry  MarkerShape=Sphere  MarkerSize=10  GraphicVisPropType=SimpleVisualProperties  GraphicDiffuseColor=[0.776470588235294, 0.756862745098039, 0.737254901960784]  GraphicSpecularColor=[0.5 0.5 0.5 1.0]  GraphicAmbientColor=[0.15 0.15 0.15 1.0]  GraphicEmissiveColor=[0.0 0.0 0.0 1.0]  GraphicShininess=75  GraphicOpacity=1
  VisualOriginTransform : sm_lib/Frames and Transforms/Rigid Transform  TranslationMethod=Cartesian  TranslationStandardOffset=0  TranslationLengthUnit=m  TranslationStandardAxis=+Z  TranslationCartesianOffset=[0, 0, 0]  TranslationROffset=0  TranslationROffsetUnits=m  TranslationZOffset=0  TranslationZOffsetUnits=m  TranslationThetaOffset=0  TranslationThetaOffsetUnits=deg  RotationMethod=RotationSequence  RotationAngleUnits=deg  RotationStandardAxis=+Z  RotationAngle=0.0  RotationArbitraryAxis=[0 0 1]  FollAlignAxisA=+X  BaseAlignAxisA=+Y  FollAlignAxisB=+Y  BaseAlignAxisB=+Z  RotationSequenceAxes=BaseAxes  RotationSequence=XYZ  RotationSequenceAngles=[0, 0, 0]  RotationSequenceAnglesUnits=rad  RotationMatrix=[1 0 0; 0 1 0; 0 0 1]
  joint3_AxisInvTransform : sm_lib/Frames and Transforms/Rigid Transform  TranslationMethod=Cartesian  TranslationStandardOffset=0  TranslationLengthUnit=m  TranslationStandardAxis=+Z  TranslationCartesianOffset=[0, 0, 0]  TranslationROffset=0  TranslationROffsetUnits=m  TranslationZOffset=0  TranslationZOffsetUnits=m  TranslationThetaOffset=0  TranslationThetaOffsetUnits=deg  RotationMethod=ArbitraryAxis  RotationAngleUnits=rad  RotationStandardAxis=+Z  RotationAngle=0  RotationArbitraryAxis=[1, 0, 0]  FollAlignAxisA=+X  BaseAlignAxisA=+Y  FollAlignAxisB=+Y  BaseAlignAxisB=+Z  RotationSequenceAxes=FollowerAxes  RotationSequence=XYX  RotationSequenceAngles=[0 0 0]  RotationSequenceAnglesUnits=deg  RotationMatrix=[1 0 0; 0 1 0; 0 0 1]
  joint4_AxisTransform : sm_lib/Frames and Transforms/Rigid Transform  TranslationMethod=Cartesian  TranslationStandardOffset=0  TranslationLengthUnit=m  TranslationStandardAxis=+Z  TranslationCartesianOffset=[0, 0, 0]  TranslationROffset=0  TranslationROffsetUnits=m  TranslationZOffset=0  TranslationZOffsetUnits=m  TranslationThetaOffset=0  TranslationThetaOffsetUnits=deg  RotationMethod=ArbitraryAxis  RotationAngleUnits=rad  RotationStandardAxis=+Z  RotationAngle=0  RotationArbitraryAxis=[1, 0, 0]  FollAlignAxisA=+X  BaseAlignAxisA=+Y  FollAlignAxisB=+Y  BaseAlignAxisB=+Z  RotationSequenceAxes=FollowerAxes  RotationSequence=XYX  RotationSequenceAngles=[0 0 0]  RotationSequenceAnglesUnits=deg  RotationMatrix=[1 0 0; 0 1 0; 0 0 1]
  joint4_OriginTransform : sm_lib/Frames and Transforms/Rigid Transform  TranslationMethod=Cartesian  TranslationStandardOffset=0  TranslationLengthUnit=m  TranslationStandardAxis=+Z  TranslationCartesianOffset=[0, 0, 0]  TranslationROffset=0  TranslationROffsetUnits=m  TranslationZOffset=0  TranslationZOffsetUnits=m  TranslationThetaOffset=0  TranslationThetaOffsetUnits=deg  RotationMethod=RotationSequence  RotationAngleUnits=deg  RotationStandardAxis=+Z  RotationAngle=0.0  RotationArbitraryAxis=[0 0 1]  FollAlignAxisA=+X  BaseAlignAxisA=+Y  FollAlignAxisB=+Y  BaseAlignAxisB=+Z  RotationSequenceAxes=BaseAxes  RotationSequence=XYZ  RotationSequenceAngles=[1.5708, 0, 1.5708]  RotationSequenceAnglesUnits=rad  RotationMatrix=[1 0 0; 0 1 0; 0 0 1]
  F : PMIOPort  Side=Left
  F1 : PMIOPort  Port=2  Side=Right
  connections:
  Inertia/RConn1 -- InertiaOriginTransform/RConn1
  ReferenceFrame/RConn1 -- InertiaOriginTransform/LConn1 -- VisualOriginTransform/LConn1 -- joint3_AxisInvTransform/LConn1 -- joint4_OriginTransform/LConn1
  Visual/RConn1 -- VisualOriginTransform/RConn1
  joint3_AxisInvTransform/RConn1 -- F/RConn1
  joint4_AxisTransform/RConn1 -- F1/RConn1
  joint4_AxisTransform/LConn1 -- joint4_OriginTransform/RConn1

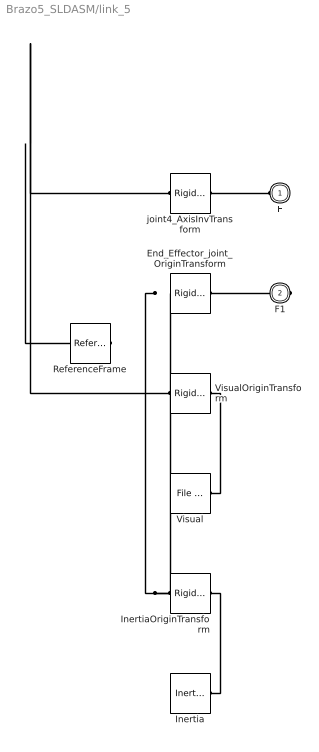
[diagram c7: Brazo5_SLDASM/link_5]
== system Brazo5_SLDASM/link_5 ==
  End_Effector_joint_OriginTransform : sm_lib/Frames and Transforms/Rigid Transform  TranslationMethod=Cartesian  TranslationStandardOffset=0  TranslationLengthUnit=m  TranslationStandardAxis=+Z  TranslationCartesianOffset=[0, 0, 0.1005]  TranslationROffset=0  TranslationROffsetUnits=m  TranslationZOffset=0  TranslationZOffsetUnits=m  TranslationThetaOffset=0  TranslationThetaOffsetUnits=deg  RotationMethod=RotationSequence  RotationAngleUnits=deg  RotationStandardAxis=+Z  RotationAngle=0.0  RotationArbitraryAxis=[0 0 1]  FollAlignAxisA=+X  BaseAlignAxisA=+Y  FollAlignAxisB=+Y  BaseAlignAxisB=+Z  RotationSequenceAxes=BaseAxes  RotationSequence=XYZ  RotationSequenceAngles=[0, 0, 0.045381]  RotationSequenceAnglesUnits=rad  RotationMatrix=[1 0 0; 0 1 0; 0 0 1]
  Inertia : sm_lib/Body Elements/Inertia  InertiaType=Custom  Mass=1.4886  MassUnits=kg  CenterOfMass=[0, 0, 0]  CenterOfMassUnits=m  MomentsOfInertia=[0.00086527, 0.00086527, 0.0015073]  MomentsOfInertiaUnits=kg*m^2  ProductsOfInertia=[-1.5349e-20, -1.2683e-19, -7.4327e-21]  ProductsOfInertiaUnits=kg*m^2  GraphicType=None  MarkerShape=Inertia  MarkerSize=20  GraphicVisPropType=SimpleVisualProperties  GraphicDiffuseColor=[0.5 0.5 0.5]  GraphicSpecularColor=[0.5 0.5 0.5 1.0]  GraphicAmbientColor=[0.15 0.15 0.15 1.0]  GraphicEmissiveColor=[0.0 0.0 0.0 1.0]  GraphicShininess=75  GraphicOpacity=1.0
  InertiaOriginTransform : sm_lib/Frames and Transforms/Rigid Transform  TranslationMethod=Cartesian  TranslationStandardOffset=0  TranslationLengthUnit=m  TranslationStandardAxis=+Z  TranslationCartesianOffset=[1.1102e-16, -1.5173e-17, 0.08550000000000001]  TranslationROffset=0  TranslationROffsetUnits=m  TranslationZOffset=0  TranslationZOffsetUnits=m  TranslationThetaOffset=0  TranslationThetaOffsetUnits=deg  RotationMethod=RotationSequence  RotationAngleUnits=deg  RotationStandardAxis=+Z  RotationAngle=0.0  RotationArbitraryAxis=[0 0 1]  FollAlignAxisA=+X  BaseAlignAxisA=+Y  FollAlignAxisB=+Y  BaseAlignAxisB=+Z  RotationSequenceAxes=BaseAxes  RotationSequence=XYZ  RotationSequenceAngles=[0, 0, 0]  RotationSequenceAnglesUnits=rad  RotationMatrix=[1 0 0; 0 1 0; 0 0 1]
  ReferenceFrame : sm_lib/Frames and Transforms/Reference Frame
  Visual : sm_lib/Body Elements/File Solid  ExtGeomFileName=Brazo5_SLDASM/meshes/link_5.STL  UnitType=Custom  ExtGeomFileUnits=m  StepReaderType=HEX  ExportConvexHullGeometry=off  InertiaType=Custom  Mass=0  MassUnits=kg  CenterOfMass=[0, 0, 0]  CenterOfMassUnits=m  MomentsOfInertia=[0, 0, 0]  MomentsOfInertiaUnits=kg*m^2  ProductsOfInertia=[0, 0, 0]  ProductsOfInertiaUnits=kg*m^2  BasedOnType=DensityFromFile  Density=1000  DensityUnits=kg/m^3  DoExposeReferenceFrame=on  SerializedFrames=<Frames/>  GraphicType=FromGeometry  MarkerShape=Sphere  MarkerSize=10  GraphicVisPropType=SimpleVisualProperties  GraphicDiffuseColor=[0.77647, 0.75686, 0.73725]  GraphicSpecularColor=[0.5 0.5 0.5 1.0]  GraphicAmbientColor=[0.15 0.15 0.15 1.0]  GraphicEmissiveColor=[0.0 0.0 0.0 1.0]  GraphicShininess=75  GraphicOpacity=1
  VisualOriginTransform : sm_lib/Frames and Transforms/Rigid Transform  TranslationMethod=Cartesian  TranslationStandardOffset=0  TranslationLengthUnit=m  TranslationStandardAxis=+Z  TranslationCartesianOffset=[0, 0, 0]  TranslationROffset=0  TranslationROffsetUnits=m  TranslationZOffset=0  TranslationZOffsetUnits=m  TranslationThetaOffset=0  TranslationThetaOffsetUnits=deg  RotationMethod=RotationSequence  RotationAngleUnits=deg  RotationStandardAxis=+Z  RotationAngle=0.0  RotationArbitraryAxis=[0 0 1]  FollAlignAxisA=+X  BaseAlignAxisA=+Y  FollAlignAxisB=+Y  BaseAlignAxisB=+Z  RotationSequenceAxes=BaseAxes  RotationSequence=XYZ  RotationSequenceAngles=[0, 0, 0]  RotationSequenceAnglesUnits=rad  RotationMatrix=[1 0 0; 0 1 0; 0 0 1]
  joint4_AxisInvTransform : sm_lib/Frames and Transforms/Rigid Transform  TranslationMethod=Cartesian  TranslationStandardOffset=0  TranslationLengthUnit=m  TranslationStandardAxis=+Z  TranslationCartesianOffset=[0, 0, 0]  TranslationROffset=0  TranslationROffsetUnits=m  TranslationZOffset=0  TranslationZOffsetUnits=m  TranslationThetaOffset=0  TranslationThetaOffsetUnits=deg  RotationMethod=ArbitraryAxis  RotationAngleUnits=rad  RotationStandardAxis=+Z  RotationAngle=0  RotationArbitraryAxis=[1, 0, 0]  FollAlignAxisA=+X  BaseAlignAxisA=+Y  FollAlignAxisB=+Y  BaseAlignAxisB=+Z  RotationSequenceAxes=FollowerAxes  RotationSequence=XYX  RotationSequenceAngles=[0 0 0]  RotationSequenceAnglesUnits=deg  RotationMatrix=[1 0 0; 0 1 0; 0 0 1]
  F : PMIOPort  Side=Left
  F1 : PMIOPort  Port=2  Side=Right
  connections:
  End_Effector_joint_OriginTransform/RConn1 -- F1/RConn1
  Inertia/RConn1 -- InertiaOriginTransform/RConn1
  InertiaOriginTransform/LConn1 -- End_Effector_joint_OriginTransform/LConn1 -- ReferenceFrame/RConn1 -- VisualOriginTransform/LConn1 -- joint4_AxisInvTransform/LConn1
  Visual/RConn1 -- VisualOriginTransform/RConn1
  joint4_AxisInvTransform/RConn1 -- F/RConn1
